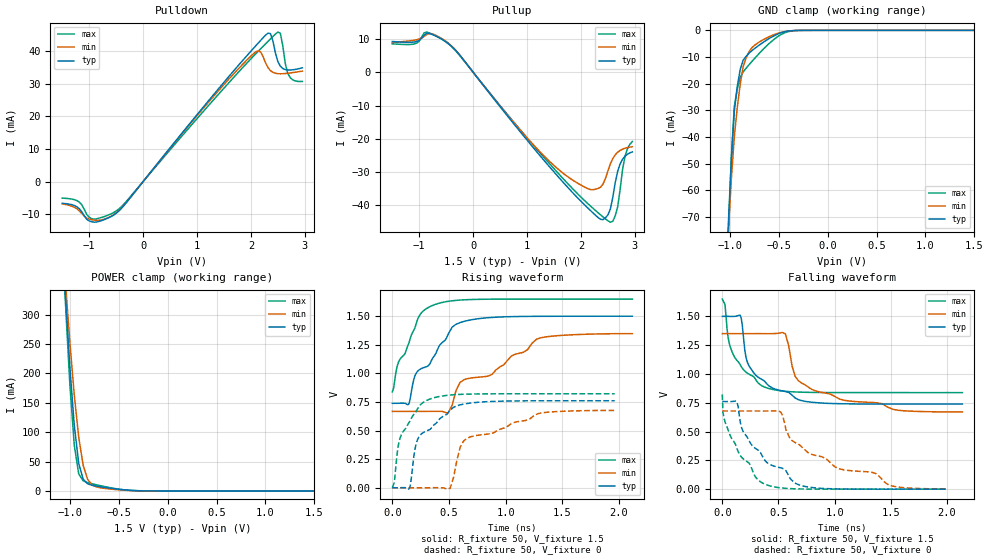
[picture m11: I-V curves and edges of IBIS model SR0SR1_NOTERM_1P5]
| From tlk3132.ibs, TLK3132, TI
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[Model]   SR0SR1_NOTERM_1P5
Model_type   3-state
Polarity   Non-Inverting
Enable   Active-Low
Cref =  15.0000pF
Rref =  100.0000M
Vref =  0V
Vmeas =  0.75
C_comp   1.311337p   1.240052p   1.381049p
[Temperature Range]   25   125   -40
[Voltage Range]   1.5   1.35   1.65
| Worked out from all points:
|   slope of the pulldown table from 0 to 0.225 V, typ, clamps not added: 48.2 ohm
|   slope of the pullup table from 0 to 0.225 V, typ, clamps not added: 48 ohm
|   GND clamp passes 1 mA (typ) near -0.48 V on its own axis
|   POWER clamp passes 1 mA (typ) near -0.38 V on its own axis
|   rising waveform, R_fixture 50, V_fixture 1.5: 20-80 % time 319ps typ, 646ps min, 200ps max; typ from 0.739 V to 1.5 V
|   rising waveform, R_fixture 50, V_fixture 0: 20-80 % time 249ps typ, 472ps min, 175ps max; typ from 0 V to 0.761 V
|   falling waveform, R_fixture 50, V_fixture 1.5: 20-80 % time 239ps typ, 402ps min, 200ps max; typ from 1.5 V to 0.739 V
|   falling waveform, R_fixture 50, V_fixture 0: 20-80 % time 415ps typ, 800ps min, 260ps max; typ from 0.761 V to 0 V
[POWER_clamp]
|   voltage   I(typ)   I(min)   I(max)
-1.5V     1.852A     1.601A     2.096A
-1.061V   377.6mA    392.9mA    374mA
-1.045V   332.8mA    356mA      321.5mA
-1.03V    292.2mA    321.8mA    275mA
-1V       211mA      253.4mA    181.9mA
-954.5mV  111.3mA    163mA      77.64mA
-909.1mV  46.83mA    91.01mA    28.92mA
-863.6mV  19.88mA    43.45mA    17.23mA
-818.2mV  12.16mA    19.6mA     14.12mA
-727.3mV  8.165mA    6.726mA    10.4mA
-409.1mV  1.376mA    880.6uA    1.274mA
1.5V      14.89nA    105.6nA    8.857nA
[Pulldown]
|   voltage   I(typ)   I(min)   I(max)
-1.5V     -6.667mA   -6.872mA   -5.079mA
-1.182V   -8.366mA   -9.005mA   -6.333mA
-954.5mV  -12.31mA   -11.68mA   -11.4mA
-454.5mV  -9.078mA   -8.982mA   -8.456mA
2.045V    40.79mA    39.16mA    38.4mA
2.182V    43.27mA    39.66mA    40.71mA
2.364V    45.32mA    33.96mA    43.74mA
2.5V      36.76mA    33.06mA    45.8mA
2.545V    35.36mA    33.02mA    45.49mA
2.682V    34.18mA    33.18mA    33.26mA
2.773V    34.24mA    33.38mA    31.19mA
2.955V    34.85mA    33.84mA    30.67mA
[Pullup]
|   voltage   I(typ)   I(min)   I(max)
-1.5V     9.208mA    8.869mA    8.526mA
-1.091V   9.066mA    9.604mA    8.486mA
-863.6mV  11.68mA    11.3mA     12.04mA
-454.5mV  8.493mA    8.644mA    8.504mA
1.727V    -34.07mA   -31.06mA   -32.95mA
2.273V    -42.98mA   -35.12mA   -41.55mA
2.409V    -44.28mA   -33.62mA   -43.43mA
2.545V    -41.14mA   -27.54mA   -45.03mA
2.636V    -33.19mA   -24.8mA    -43.12mA
2.727V    -27.53mA   -23.48mA   -35.21mA
2.818V    -25.23mA   -22.82mA   -25.22mA
2.955V    -23.93mA   -22.38mA   -20.79mA
[GND_clamp]
|   voltage   I(typ)   I(min)   I(max)
-1.5V     -1.99A     -1.518A    -2.426A
-1.015V   -72.36mA   -74.91mA   -76.76mA
-984.8mV  -48.51mA   -55.8mA    -47.87mA
-954.5mV  -30.42mA   -39.97mA   -28.58mA
-924.2mV  -21.06mA   -28.95mA   -21.99mA
-893.9mV  -14.64mA   -20.14mA   -17.66mA
-863.6mV  -11.15mA   -13.54mA   -15.57mA
-803mV    -8.521mA   -7.949mA   -12.86mA
-712.1mV  -5.867mA   -4.684mA   -9.137mA
-500mV    -1.209mA   -994.1uA   -2.074mA
-348.5mV  -89.2uA    -110.3uA   -156.7uA
1.5V      14.89nA    6.861uA    -6.796nA
[Ramp]
| variable   typ   min   max
dV/dt_f  0.4634222/0.2350662n  0.4152239/0.4029393n  0.4921042/0.197383n
dV/dt_r  0.4640071/0.246391n   0.4159768/0.4730128n  0.4989111/0.1746655n
R_load = 50
[Rising Waveform]
R_fixture = 50
V_fixture = 1.5
V_fixture_min = 1.35
V_fixture_max = 1.65
|   time   V(typ)   V(min)   V(max)
0s        738.5mV    668mV      838.2mV
48ps      738.7mV    668mV      1.08V
144ps     729.5mV    668mV      1.259V
237ps     1.031V     668mV      1.501V
372ps     1.155V     668.6mV    1.601V
492ps     1.34V      654.2mV    1.63V
597ps     1.444V     920.7mV    1.641V
879ps     1.489V     990.9mV    1.649V
1.272ns   1.499V     1.298V     1.65V
2.118ns   1.5V       1.347V     1.65V
[Rising Waveform]
R_fixture = 50
V_fixture = 0
V_fixture_min = 0
V_fixture_max = 0
|   time   V(typ)   V(min)   V(max)
0s        43.28uV    35.23uV    48.88uV
78ps      966.3uV    34.92uV    459.9mV
147ps     -10.86mV   35.92uV    569mV
213ps     393.4mV    37.77uV    670.6mV
321ps     504.8mV    197.9uV    771.5mV
510ps     678.1mV    -5.429mV   810.8mV
600ps     725.2mV    357.4mV    816.6mV
660ps     736.6mV    433.3mV    818.7mV
1.296ns   760.5mV    650.6mV    822.1mV
1.962ns   760.9mV    675.9mV    822.1mV
[Falling Waveform]
R_fixture = 50
V_fixture = 1.5
V_fixture_min = 1.35
V_fixture_max = 1.65
|   time   V(typ)   V(min)   V(max)
0s        1.5V       1.35V      1.65V
99ps      1.499V     1.35V      1.166V
168ps     1.488V     1.35V      1.065V
201ps     1.202V     1.35V      1.024V
237ps     1.072V     1.35V      998.8mV
378ps     935.3mV    1.35V      885.6mV
561ps     847.6mV    1.35V      849.5mV
648ps     791.5mV    979.8mV    843.9mV
822ps     752.1mV    855.4mV    839.6mV
2.136ns   738.6mV    670.7mV    838.2mV
[Falling Waveform]
R_fixture = 50
V_fixture = 0
V_fixture_min = 0
V_fixture_max = 0
|   time   V(typ)   V(min)   V(max)
0s        760.9mV    678.6mV    822.1mV
15ps      761mV      678.6mV    617.5mV
72ps      760.4mV    678.6mV    461.1mV
129ps     760.9mV    678.6mV    358mV
186ps     500.3mV    678.6mV    263.3mV
384ps     244mV      678.3mV    41.8mV
522ps     184.6mV    666.6mV    10.99mV
687ps     35.35mV    384.9mV    2.082mV
1.041ns   1.924mV    176.8mV    95.59uV
1.989ns   44.38uV    2.782mV    49.1uV
